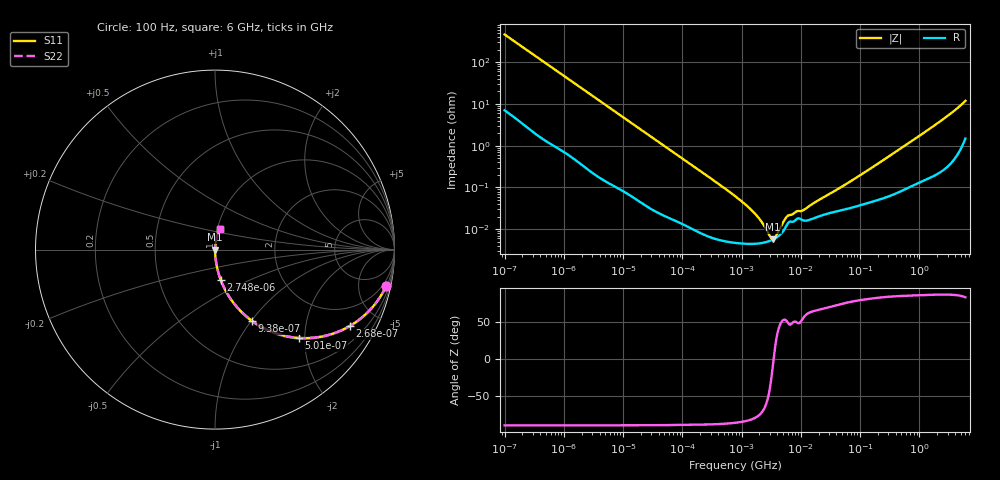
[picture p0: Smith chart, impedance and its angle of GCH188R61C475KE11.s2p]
!Murata Part Number: GCH188R61C475KE11
!These Parameters are Measured in Series Mode Connection
!Data Generated on Mar 13, 2026
!  o--ll--o
!Port1  Port2
!  o------o
!Operation Temp=25[degC], DC Bias Voltage=0[V]
!Freq. Start=100[Hz] Stop=6[GHz] 401[Steps]
# Hz S RI R 50
!Freq.(Hz) S11(Real) S11(Imag) S21(Real) S21(Imag) S12(Real) S12(Imag) S22(Real) S22(Imag)
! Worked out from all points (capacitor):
!   401 points, 100 Hz to 6 GHz, reference 50 ohm
!   read as one part in series: C = 3.43 uF near 109 Hz
!   lowest |Z| = 5.7 mohm at 3.394 MHz (marker M1)
!   series resonance near 3.476 MHz, so ESL is about 610 pH
!   S11 on the Smith chart (normalised r, x): 100 Hz: 1.14, -9.25; 268 Hz: 1.05, -3.49; 501 Hz: 1.03, -1.87; 938 Hz: 1.01, -1.01; 2.748 kHz: 1.00, -0.35; 6 GHz: 1.03, +0.24
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100  0.9525 -0.2052  0.0475 0.2052  0.0475 0.2052  0.9525 -0.2052
164  0.8862 -0.3102  0.1138 0.3102  0.1138 0.3102  0.8862 -0.3102
268  0.7496 -0.4263  0.2504 0.4263  0.2504 0.4263  0.7496 -0.4263
501  0.4675 -0.4921  0.5325 0.4921  0.5325 0.4921  0.4675 -0.4921
938  0.2054 -0.3966  0.7946 0.3966  0.7946 0.3966  0.2054 -0.3966
2008  0.056 -0.2228  0.944 0.2228  0.944 0.2228  0.056 -0.2228
2748  0.0315 -0.1677  0.9685 0.1677  0.9685 0.1677  0.0315 -0.1677
8047  0.00452 -0.0594  0.9955 0.0594  0.9955 0.0594  0.00452 -0.0594
40335  0.000387 -0.0121  0.9996 0.0121  0.9996 0.0121  0.000387 -0.0121
774597  4.74e-05 -0.000621  1 0.000621  1 0.000621  4.74e-05 -0.000621
1585629  4.46e-05 -0.000255  1 0.000255  1 0.000255  4.46e-05 -0.000255
2594782  4.92e-05 -8.76e-05  1 8.76e-05  1 8.76e-05  4.92e-05 -8.76e-05
3394479  5.66e-05 -7e-06  0.9999 7e-06  0.9999 7e-06  5.66e-05 -7e-06
4246196  6.93e-05 6.12e-05  0.9999 -6.12e-05  0.9999 -6.12e-05  6.93e-05 6.12e-05
6075234  0.00014 0.000159  0.9999 -0.000159  0.9999 -0.000159  0.00014 0.000159
8692127  0.000179 0.000204  0.9998 -0.000204  0.9998 -0.000204  0.000179 0.000204
1.087309e7  0.000163 0.00023  0.9998 -0.00023  0.9998 -0.00023  0.000163 0.00023
1.555665e7  0.000177 0.000359  0.9998 -0.000359  0.9998 -0.000359  0.000177 0.000359
6.233367e7  0.000312 0.00124  0.9997 -0.00124  0.9997 -0.00124  0.000312 0.00124
3.124326e8  0.000651 0.00561  0.9993 -0.00561  0.9993 -0.00561  0.000651 0.00561
2.142435e9  0.00351 0.0362  0.9965 -0.0362  0.9965 -0.0362  0.00351 0.0362
6e9  0.0279 0.1133  0.9721 -0.1133  0.9721 -0.1133  0.0279 0.1133
